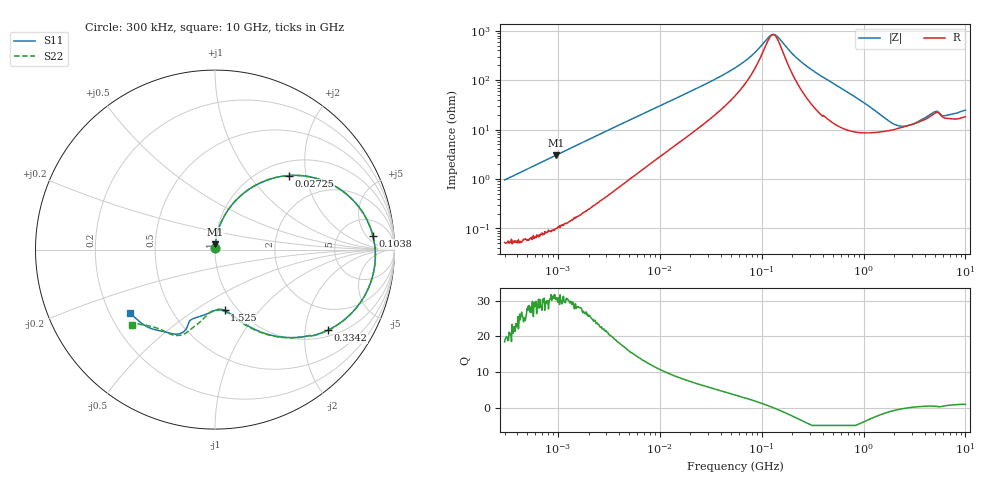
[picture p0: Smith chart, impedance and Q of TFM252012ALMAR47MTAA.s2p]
! S-Parameter Data Generated by TDK Corporation
! Copyright(C) 2019 TDK Corporation.
! All Rights Reserved.
! TDK P/N: TFM252012ALMAR47MTAA (Inductor)
! Property: L=470nH at 1MHz
! Size(LxWxT): 2.5x2x1.2mm
! Model Type: s2p (Touchstone File Format Version 1.0)
! Frequency: DC=Yes Start=0.3MHz Stop=10000MHz 802points Log-sweep
! Model Generated on May 10, 2019
! Port Assignments:
!  1 ---@@@--- 2
! Applicable Conditions:
!  Temperature = 25 degC
!  DC Bias Current = 0 A
!  Small Signal Operation
! Terms and conditions regarding TDK Simulation Models
! (1)This simulation model is being provided solely for informational purposes. Please refer to the specifications of the products in terms of detailed characteristics of such products.
! (2)In no event shall TDK Corporation of any of its subsidiaries be liable for any loss or damage arising, directly or indirectly,
!  From any information contained in this simulation model, including, but not limited to loss or damages arising from any inaccuracies, omissions or errors in connection with such information.
! (3)Any and all copyrights on this simulation model are owned by TDK Corporation.
!  Duplication or redistribution of this simulation model without prior written permission from TDK Corporation is prohibited.
! (4)This simulation model is subject to any modification or change without any prior notice.
! (5)Neither TDK Corporation nor any of its subsidiaries shall make any warranty, express or implied,
!  Including but not limited to the correctness, implied warranties of merchantability and fitness for a particular purpose with respect to this simulation models.
! (6)The use of this simulation model shall be deemed to have consented to the terms and conditions hereof.
# Hz S MA R 50
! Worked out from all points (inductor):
!   801 points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, 300 kHz to 10 GHz, reference 50 ohm
!   read as one part in series: L = 505 nH near 318.3 kHz
!   highest Q = 31 at 954.6 kHz (marker M1), where L = 503 nH
!   self-resonance near 129.4 MHz
!   S11 on the Smith chart (normalised r, x): 300 kHz: 1.00, +0.02; 27.25 MHz: 1.28, +1.60; 103.8 MHz: 11, +8; 334.2 MHz: 1.19, -2.66; 1.525 GHz: 0.87, -0.67; 10 GHz: 0.28, -0.31
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300000  0.009551 87.2  0.9993 -0.5  0.9992 -0.5  0.009822 87.8
954628  0.03003 86.4  0.9985 -1.7  0.9986 -1.7  0.03017 86.4
1713600  0.05355 84.8  0.9967 -3.1  0.9966 -3.1  0.0536 84.8
9671944  0.2734 68.8  0.9371 -15.9  0.9372 -15.9  0.2734 68.8
2.725275e7  0.5826 45.1  0.7232 -35.5  0.7232 -35.5  0.5825 45.1
5.477226e7  0.7838 24.4  0.4433 -49.8  0.4433 -49.8  0.7838 24.4
8.035641e7  0.8551 12.8  0.2683 -51.8  0.2683 -51.8  0.8552 12.8
1.038383e8  0.8833 4.9  0.1581 -40.9  0.1581 -40.9  0.8834 4.9
1.226455e8  0.8926 -0.3  0.1105 -14.8  0.1105 -14.8  0.8927 -0.3
1.356511e8  0.8946 -3.5  0.108 9.9  0.108 9.9  0.8946 -3.6
2.039737e8  0.8723 -17.2  0.2622 50.9  0.2622 50.9  0.8723 -17.3
3.126428e8  0.7916 -32.9  0.4784 46.1  0.4784 46.1  0.7917 -33.0
3.342219e8  0.7736 -35.4  0.5111 44.3  0.5111 44.3  0.7738 -35.5
4.986356e8  0.6411 -49.8  0.6781 31.7  0.6782 31.7  0.6417 -50.0
7.497801e8  0.4986 -63.4  0.7936 18.0  0.7936 17.9  0.4995 -63.6
1.525386e9  0.3424 -80.9  0.8582 -4.9  0.8582 -4.9  0.3449 -82.0
1.767019e9  0.334 -84.4  0.8558 -9.6  0.8558 -9.6  0.3371 -85.8
2.659614e9  0.3516 -94.3  0.8261 -23.1  0.8262 -23.1  0.3582 -95.6
4.22443e9  0.413 -108.8  0.7435 -40.8  0.7436 -40.8  0.4399 -104.7
5.849356e9  0.5241 -116.3  0.6597 -50.5  0.6597 -50.5  0.5338 -118.8
8.09931e9  0.5792 -134.6  0.5924 -70.3  0.5923 -70.3  0.5983 -136.3
1e10  0.5908 -143.0  0.5346 -81.8  0.5347 -81.8  0.6258 -137.6
